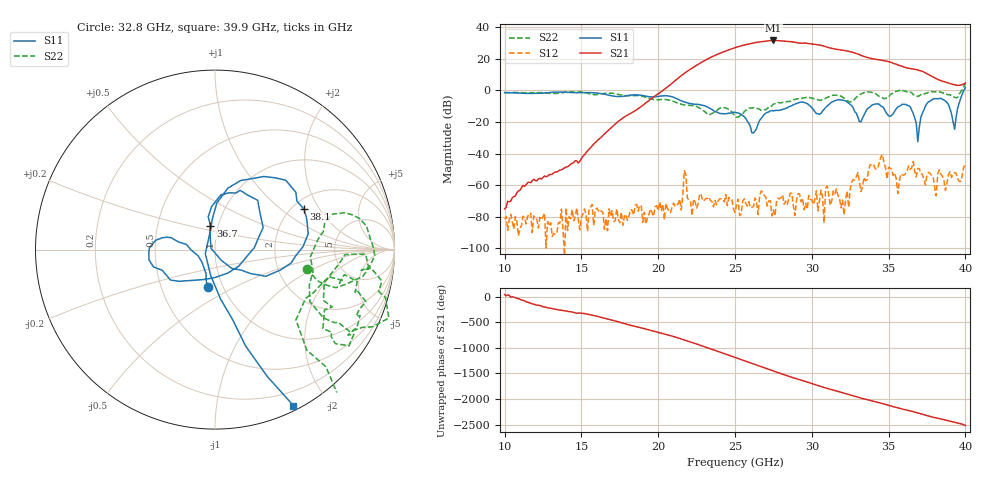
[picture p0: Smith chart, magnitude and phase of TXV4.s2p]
!Keysight Technologies,M9808A,MY58100618,A.14.70.03
!Date: Monday, February 27, 2023 13:37:44
!Correction: S11(C  2-Port  )
!S21(C  2-Port  )
!S12(C  2-Port  )
!S22(C  2-Port  )
!S2P File: Measurements: S11, S21, S12, S22:
# Hz S  RI  R 50
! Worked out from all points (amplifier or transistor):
!   301 points, 10 GHz to 40 GHz, reference 50 ohm
!   highest |S21| = 31.4 dB at 27.5 GHz (marker M1)
!   |S21| within 3 dB of that: 25.56 GHz to 30.56 GHz (4.997 GHz wide, 17.8 % of centre)
!   unconditionally stable (mu >= 1): start of sweep to 35.72 GHz; 35.9 GHz to 39.77 GHz
!   at 15 GHz: K = 43951.49, MAG = -30.8 dB, |S12| = -80.3 dB
!   at 25 GHz: K = 154.71, MAG = 27.2 dB, |S12| = -77.3 dB
!   at 40 GHz: K = 64.70, MSG = 26.2 dB, |S12| = -47.9 dB
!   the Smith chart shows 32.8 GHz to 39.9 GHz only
!   S11 on the Smith chart (normalised r, x): 32.8 GHz: 0.86, -0.37; 36.7 GHz: 0.92, +0.25; 38.1 GHz: 2.31, +1.47; 39.9 GHz: 0.05, -1.62
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1e10  0.7228 0.4283  0.000126 0.000125  -8.1e-05 -2.6e-05  0.1316 0.8223
1.5e10  0.6337 -0.5453  0.00535 0.00448  9.57e-05 -1.06e-05  0.6774 0.5873
2e10  -0.2179 -0.5976  0.7089 0.3074  -0.000157 -8.79e-07  0.2122 -0.4481
2.34e10  -0.2557 -0.0616  4.98 9.626  -0.000248 -0.000214  -0.0845 -0.1509
2.42e10  -0.1711 0.0621  14.79 -5.834  -2.82e-05 -0.000353  -0.2054 -0.1905
2.5e10  -0.1381 0.1428  -5.868 -21.29  -3.69e-06 -0.000137  -0.1328 -0.0961
2.58e10  -0.0576 0.0884  -27.6 5.487  0.000171 -0.000139  -0.2256 0.106
2.65e10  0.0853 -0.00862  -2.744 32.91  7.37e-05 9.3e-05  -0.2252 0.1356
2.69e10  0.1609 -0.0634  21.58 27.69  0.000455 -9.63e-05  -0.1408 0.1977
2.75e10  0.184 -0.1245  36.44 -8.098  3.43e-05 -0.000162  -0.0436 0.3581
2.82e10  0.1092 -0.2309  2.606 -35.61  -3.65e-06 0.000249  0.0162 0.4199
2.89e10  0.036 -0.363  -29.63 -13.66  0.00011 1.25e-05  0.1943 0.4687
2.95e10  0.0712 -0.4038  -26.99 15  0.00011 0.000125  0.1663 0.5503
3e10  0.0651 -0.2744  -5.816 28.32  -0.000326 9.69e-05  0.1493 0.5487
3.1e10  -0.2643 -0.1688  22.82 2.638  0.000419 0.000846  0.4902 0.3236
3.19e10  -0.2669 -0.4142  6.673 -17.53  -7.63e-05 -0.000176  0.4866 0.4329
3.28e10  -0.0373 -0.2058  -12.9 -7.775  0.000218 -0.00142  0.5126 -0.1055
3.5e10  -0.00345 -0.1565  6.472 4.616  9.76e-05 0.00363  0.5285 -0.2902
3.67e10  -0.0252 0.1321  -0.5472 -4.522  0.00116 -0.00255  0.6894 -0.0824
3.81e10  0.496 0.2244  -1.977 1.187  -0.000105 -0.000445  0.8087 -0.3675
3.99e10  0.4365 -0.8687  1.527 0.4022  -0.00156 -0.00353  0.8049 -1.046
4e10  0.5766 -1.097  1.696 0.0401  0.00288 -0.00285  1.036 -1.267
